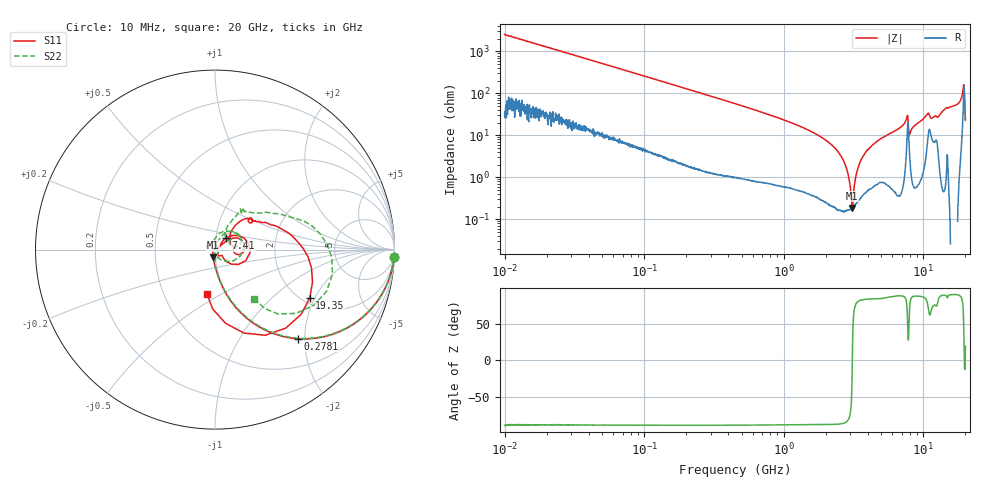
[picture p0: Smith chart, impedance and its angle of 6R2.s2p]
!Keysight Technologies,P5008B,MY61100088,A.16.20.02
!Date: Monday, November 06, 2023 15:50:07
!Correction: S11(C  2-Port  )
!S21(C  2-Port  )
!S12(C  2-Port  )
!S22(C  2-Port  )
!S2P File: Measurements: S11, S21, S12, S22:Log Frequency Sweep
# Hz S  dB  R 50
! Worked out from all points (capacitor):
!   1601 points, 10 MHz to 20 GHz, reference 50 ohm
!   read as one part in series: C = 6.27 pF near 10.39 MHz
!   lowest |Z| = 187 mohm at 3.092 GHz (marker M1)
!   series resonance near 3.096 GHz, so ESL is about 420 pH
!   S11 on the Smith chart (normalised r, x): 10 MHz: 2, -50; 278.1 MHz: 1.01, -1.85; 7.41 GHz: 1.12, +0.14; 19.35 GHz: 2.19, -1.83; 20 GHz: 0.81, -0.43
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1e7  -0.01 -2.3  -28.11 87.0  -28.11 87.0  -0.01 -2.3
3.555162e7  -0.11 -7.9  -17.34 80.9  -17.34 80.9  -0.11 -7.9
1.263918e8  -0.97 -26.0  -7.24 63.1  -7.24 63.1  -0.98 -25.9
2.780998e8  -3.37 -47.1  -2.79 42.2  -2.79 42.2  -3.39 -46.8
4.472136e8  -6.06 -60.1  -1.32 29.1  -1.32 29.1  -6.10 -59.8
1.589917e9  -16.77 -83.5  -0.14 5.6  -0.15 5.6  -17.13 -84.5
3.091822e9  -26.96 -106.1  -0.06 -2.6  -0.06 -2.6  -26.07 -85.6
4.170543e9  -38.19 -143.1  -0.05 -6.7  -0.06 -6.7  -32.46 -48.6
4.71883e9  -49.64 151.9  -0.05 -8.5  -0.06 -8.5  -34.73 -11.2
5.652411e9  -38.24 40.4  -0.05 -11.5  -0.05 -11.5  -33.84 61.7
7.410252e9  -21.02 46.0  -0.19 -19.3  -0.20 -19.3  -21.53 79.1
7.770776e9  -14.76 -19.4  -1.61 -14.8  -1.61 -14.8  -16.69 -13.9
8.187644e9  -34.47 -36.9  -0.11 -16.3  -0.11 -16.3  -38.49 -101.0
8.464494e9  -34.82 20.5  -0.06 -18.0  -0.06 -18.1  -46.19 107.8
9.132954e9  -27.76 35.9  -0.04 -21.1  -0.05 -21.1  -31.07 80.0
1.068304e10  -16.60 24.2  -0.60 -29.4  -0.61 -29.4  -16.87 44.0
1.249622e10  -19.21 7.8  -0.64 -26.8  -0.64 -26.8  -20.21 31.6
1.434201e10  -12.20 44.7  -0.25 -36.3  -0.25 -36.3  -12.26 57.7
1.767617e10  -10.79 32.8  -0.52 -52.2  -0.53 -52.2  -10.67 44.5
1.853616e10  -8.33 17.9  -1.16 -61.8  -1.17 -61.8  -8.04 30.4
1.934586e10  -4.54 -27.1  -6.29 -71.5  -6.29 -71.5  -3.70 -4.1
2e10  -12.06 -100.3  -2.29 -26.4  -2.29 -26.5  -9.13 -51.3
